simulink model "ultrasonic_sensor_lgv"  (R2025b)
settings: Solver=FixedStepAuto  StartTime=0.0  StopTime=inf  RelTol=1e-3  EnableMultiTasking=on
libraries: arduinosensorlib x1

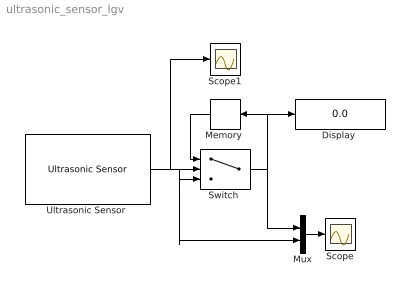
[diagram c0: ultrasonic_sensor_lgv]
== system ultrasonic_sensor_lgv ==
  "Display " : Display
  "Memory " : Memory
  Mux : Mux  Inputs=2
  Scope : Scope
  Scope1 : Scope
  "Switch " : Switch  Criteria=u2 > Threshold  Threshold=0.1
  "Ultrasonic Sensor " : arduinosensorlib/Ultrasonic Sensor  NumSignalPins=2  TrigPin=4  EchoPin=5  SignalPin=3  SampleTime_=0.01  blockPlatform=ARDUINO
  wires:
  "Ultrasonic Sensor "/1 -> Scope1/1, "Switch "/3, Mux/2, "Switch "/2
  "Memory "/1 -> "Switch "/1
  "Switch "/1 -> Mux/1, "Display "/1, "Memory "/1
  Mux/1 -> Scope/1
